PROGRAM MAIN

VAR CONSTANT	
    cInitSource			: ST_MA_MultiArray_InitPars := ( eTypeCode := eMA_TypeCode_LREAL, nDims := 1, aDimSizes := [cBufferLength]);	
END_VAR

VAR
	// Signal generation (summed up sine wave)
	fSetFrequency 		: ARRAY[1..9] OF LREAL := [100, 500, 700, 900, 1100, 1400, 1800, 2300, 2800];		// devided by 0.001 in signal generatrion
	fSetAmplitude		: ARRAY[1..9] OF LREAL := [-3.5, 4 , -8 , 6 , -4 ,-8 ,6 , -8];						// amplitudes of signal parts [defined in MPa, see GVL_constants]
	fDC					: LREAL := 0.0;
	
 	fbFunctionGenerator	: ARRAY[1..9] OF FB_FunctionGenerator;
	aBufferSignal		: ARRAY[1..cOversamples] OF LREAL;  // signal part
	aBuffer				: ARRAY[1..cOversamples] OF LREAL;  // sum of signals

	// Read signal from file
	bBufferFull			: BOOL := TRUE;
	fbReadCsvFile		: FB_CMA_ReadCsvFile := (bExecute:=TRUE, sSeparator:=';', sFileName:='C:\DCSine.csv', nHeaderLines := 6);
	nLastErrorId		: UDINT;
	nFullBufferCount	: UDINT;
							
	// Input selection
	nInputSelection		: UDINT := 1;						// Switch between hardware and function generator	
	nSample				: UDINT;
	Iter				: UDINT;
	aLoadInput AT %I*	: ARRAY[1..cOversamples] OF DINT;	// Input from hardware e.g. ELM35xx

	// Input/Output
	fbSource			: FB_CMA_Source :=(	stInitPars := cInitSource, nOwnID := eID_Source, aDestIDs := [eID_RainflowCounting]);	// Initialize source buffers
	fbSink_MR_RFC		: FB_CMA_Sink := (nOwnID := eID_Sink_MR_RFC);
	fbSink_MR_MSC		: FB_CMA_Sink := (nOwnID := eID_Sink_MR_MSC);

	// Results from Miners Rule, i.e. [ damage, halfcycles ]
	aResults_RFC		: ARRAY[0..1] OF LREAL;
	aResults_MSC		: ARRAY[0..1] OF LREAL;
	
	// Damage prediction (by Miners rule)
	bResetDamage		: BOOL := TRUE;			// Reset base damage.
	bInitDamage			: BOOL := TRUE;			// Initialize base damage.
	fBaseDamage_RFC		: LREAL;				// Base damage of Rainflow counting from previous runs, additive to result of online value.								
	fBaseDamage_MSC		: LREAL;				// Base damage of mean stress corrected Rainflow counting from previous runs, additive to result of online value.
	fDamage_RFC			: LREAL;				// Damage calculated based on Rainflow counting.
	fDamage_MSC			: LREAL;				// Damage calculated based on mean stress corrected Rainflow counting.
	nBaseCycles_RFC		: ULINT;				// Initial number of cycles of Rainflow counting from previous runs, additive to result of online value.							               
	nBaseCycles_MSC		: ULINT;	            // Initial number of cycles of mean stress corrected Rainflow counting from previous runs, additive to result of online value.
	nCycles_RFC			: ULINT;				// Number of (half) cycles counted; Rainflow counting only.
	nCycles_MSC			: ULINT;				// Number of (half) cycles counted; mean stress corrected Rainflow counting.
	
	// Info levels
	fWarning			: LREAL := 0.7;			// Warning level at 70%
	fCritical			: LREAL := 0.9;			// Critical level at 90%
	fError				: LREAL := 1.0;			// predicted Error level at 100% (end of lifetime)
	
	// Propagation of lifetime
	tTimeStampStart		: ULINT;				// in 100ns
	tLifetime_RFC		: LREAL;				// Lifetime in seconds
	tLifetime_MSC		: LREAL;				// Lifetime in seconds
	
	// Status and error handling
	bAnalysisStarted	: BOOL := FALSE;
	bStartTrigger		: BOOL := FALSE;
	bCalculate			: BOOL;
	fbErrHist			: FB_HRErrHist; 		// error monitoring
	
	// local vars
	hr					: HRESULT;
	n,m					: UDINT;
END_VAR

IF NOT bAnalysisStarted THEN
	tTimeStampStart := F_GetTaskTime();
	bAnalysisStarted := TRUE;
END_IF
IF NOT bStartTrigger THEN
	bStartTrigger := TRUE;
ELSE
	bStartTrigger := FALSE;
END_IF

// what to do if persistent data from is available at TwinCAT Satup? 
// Use case: Application is running for a time frame. IPC has to restart, e.g. for service.
// Persistent data ensures that counting continous and is not reset to zero. 
IF bInitDamage THEN
	IF bResetDamage THEN
		GVL_Persistant.fDamage_RFC := 0.0;
		GVL_Persistant.fDamage_MSC := 0.0;
		GVL_Persistant.nCycles_RFC := 0;
		GVL_Persistant.nCycles_MSC := 0;
		bResetDamage := FALSE;
	END_IF
	fBaseDamage_RFC := GVL_Persistant.fDamage_RFC;
	fBaseDamage_MSC := GVL_Persistant.fDamage_MSC;
	nBaseCycles_RFC := GVL_Persistant.nCycles_RFC;
	nBaseCycles_MSC := GVL_Persistant.nCycles_MSC;
	bInitDamage := FALSE;
END_IF


// input signal for fatigue damaga analysis 
// from terminal, from signal generator or from file
CASE nInputSelection OF
	0:  (* input from ELM35xx (SG Terminal) *)
		FOR nSample := 1 TO cOversamples DO
			aBuffer[nSample] := DINT_TO_LREAL(aLoadInput[nSample]);
			//aBuffer[nSample] := c * aBuffer[nSample] with c being scale to convert raw input to MPa (Young's modulus, measurement range, k factor)
		END_FOR
	1:  (* signal generator => generates a synthetik stress signal*)		
		FOR nSample := 1 TO cOversamples DO
			aBuffer[nSample] := 0;
		END_FOR
		FOR Iter := 1 TO 9 DO
			fbFunctionGenerator[Iter](	fFrequency 	:= 0.001 * fSetFrequency[Iter],
										fAmplitude 	:= fSetAmplitude[Iter],
										eFunction 	:= E_FunctionType.Sine,
										aSignal		:= aBufferSignal );
									
			FOR nSample := 1 TO cOversamples DO
				aBuffer[nSample] := aBuffer [nSample] + aBufferSignal[nSample] + fDC;
			END_FOR
		END_FOR
	2: (* Data from file *)
		bBufferFull := FALSE;
		IF NOT fbReadCsvFile.bError THEN
			fbReadCsvFile(aBuffer := aBuffer, bBufferFull => bBufferFull);
			IF fbReadCsvFile.bError THEN
				hr := fbReadCsvFile.hrErrorCode;
			END_IF
			IF bBufferFull THEN
				nFullBufferCount := nFullBufferCount + 1;
			END_IF
		ELSE
			FOR nSample := 1 TO cOversamples DO
				aBuffer[nSample] := aBuffer[cOversamples];
			END_FOR
			bBufferFull := TRUE;
		END_IF
END_CASE	

// Call source to collect data
CollectData();

// Collect results
CollectResults();

METHOD CollectData : BOOL
VAR_INPUT
END_VAR
// Call source to collect data
IF bBufferFull THEN
	fbSource.Input1DStd(pDataIn 		:= ADR(aBuffer),
						nDataInSize 	:= SIZEOF(aBuffer), 
						eElementType 	:= eMA_TypeCode_LREAL,
						nOptionPars		:= cCMA_Option_MarkInterruption); 
	IF fbSource.bError THEN
		fbErrHist.AddError(bErr:=TRUE, hrErrCode:=fbSource.hrErrorCode, sErrSource:='MAIN.fbSource'); // error monitoring
		// ToDo: if error
	END_IF
END_IF
END_METHOD

METHOD CollectResults : BOOL
VAR_INPUT
END_VAR
VAR
	fbGetTaskIdx	: GETCURTASKINDEX;
END_VAR
(* Damage calculation without Mean-stress correction *)

// Push results to sink
fbSink_MR_RFC.Output1DStd(	pDataOut 		:= ADR(aResults_RFC), 
							nDataOutSize 	:= SIZEOF(aResults_RFC), 
							eElementType 	:= eMA_TypeCode_LREAL, 	
							nOptionPars 	:= 0,			
							bNewResult		=> bCalculate );

IF fbSink_MR_RFC.bError THEN
	fbErrHist.AddError(bErr:=TRUE, hrErrCode:=fbSink_MR_RFC.hrErrorCode, sErrSource:='MAIN.fbSink_MR_RFC'); // error monitoring
	// ToDo: if error
END_IF

IF bCalculate THEN
	// Accumulate damage
	fDamage_RFC := aResults_RFC[0] + fBaseDamage_RFC;
	nCycles_RFC := LREAL_TO_ULINT(aResults_RFC[1]) + nBaseCycles_RFC;
	
	// Calculate remaining lifetime.
	IF fDamage_RFC <> fBaseDamage_RFC AND fDamage_RFC <> GVL_Persistant.fDamage_RFC THEN
		tLifetime_RFC := 1E-7 * ULINT_TO_LREAL((F_GetTaskTime() - tTimeStampStart)) * (1.0 - fDamage_RFC) / (fDamage_RFC - fBaseDamage_RFC);
	END_IF
	
	// update persistant variable
	GVL_Persistant.fDamage_RFC := fDamage_RFC;
	GVL_Persistant.nCycles_RFC := nCycles_RFC;
END_IF

(* Damage calculation with Mean-stress correction *)

// Push results to sink
fbSink_MR_MSC.Output1DStd(	pDataOut 		:= ADR(aResults_MSC), 
							nDataOutSize 	:= SIZEOF(aResults_MSC), 
							eElementType 	:= eMA_TypeCode_LREAL, 	
							nOptionPars 	:= 0,			
							bNewResult		=> bCalculate );

IF fbSink_MR_MSC.bError THEN
	fbErrHist.AddError(bErr:=TRUE, hrErrCode:=fbSink_MR_MSC.hrErrorCode, sErrSource:='MAIN.fbSink_MR_MSC'); // error monitoring
	// ToDo: if error
END_IF

IF bCalculate THEN
	// Accumulate damage
	fDamage_MSC := aResults_MSC[0] + fBaseDamage_MSC;
	nCycles_MSC := LREAL_TO_ULINT(aResults_MSC[1]) + nBaseCycles_MSC;
	
	// Calculate remaining lifetime.
	IF fDamage_MSC <> fBaseDamage_MSC AND fDamage_MSC <> GVL_Persistant.fDamage_MSC THEN
		tLifetime_MSC := 1E-7 * ULINT_TO_LREAL((F_GetTaskTime() - tTimeStampStart)) * (1.0 - fDamage_MSC) / (fDamage_MSC - fBaseDamage_MSC);
	END_IF
	
	// update persistant variable
	GVL_Persistant.fDamage_MSC := fDamage_MSC;
	GVL_Persistant.nCycles_MSC := nCycles_MSC;
END_IF
END_METHOD

END_PROGRAM
